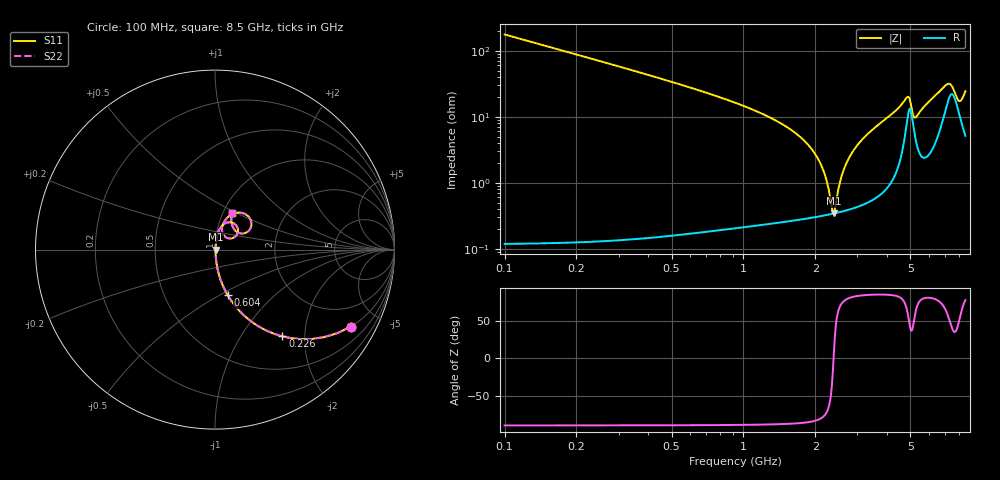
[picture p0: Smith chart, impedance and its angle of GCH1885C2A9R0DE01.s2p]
!Murata Part Number: GCH1885C2A9R0DE01
!These Parameters are Measured in Series Mode Connection
!Data Generated on Mar 13, 2026
!  o--ll--o
!Port1  Port2
!  o------o
!Operation Temp=25[degC], DC Bias Voltage=0[V]
!Freq. Start=100[MHz] Stop=9[GHz] 401[Steps]
# Hz S RI R 50
!Freq.(Hz) S11(Real) S11(Imag) S21(Real) S21(Imag) S12(Real) S12(Imag) S22(Real) S22(Imag)
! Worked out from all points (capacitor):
!   401 points, 100 MHz to 8.5 GHz, reference 50 ohm
!   read as one part in series: C = 9 pF near 142 MHz
!   lowest |Z| = 343 mohm at 2.389 GHz (marker M1)
!   series resonance near 2.385 GHz, so ESL is about 490 pH
!   S11 on the Smith chart (normalised r, x): 100 MHz: 1.00, -3.53; 226 MHz: 1.00, -1.55; 604 MHz: 1.00, -0.55; 8.5 GHz: 1.10, +0.48
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1e8  0.7569 -0.4286  0.2431 0.4286  0.2431 0.4286  0.7569 -0.4286
2.26e8  0.3757 -0.4835  0.6243 0.4835  0.6243 0.4835  0.3757 -0.4835
3.73e8  0.177 -0.3801  0.823 0.3801  0.823 0.3801  0.177 -0.3801
6.04e8  0.0713 -0.2542  0.9287 0.2542  0.9287 0.2542  0.0713 -0.2542
1.507e9  0.00758 -0.0706  0.9924 0.0706  0.9924 0.0706  0.00758 -0.0706
1.843e9  0.0044 -0.0391  0.9956 0.0391  0.9956 0.0391  0.0044 -0.0391
2.074e9  0.00353 -0.0212  0.9965 0.0212  0.9965 0.0212  0.00353 -0.0212
2.2e9  0.00336 -0.0123  0.9966 0.0123  0.9966 0.0123  0.00336 -0.0123
2.347e9  0.00337 -0.00244  0.9966 0.00244  0.9966 0.00244  0.00337 -0.00244
2.389e9  0.00341 0.00027  0.9966 -0.00027  0.9966 -0.00027  0.00341 0.00027
2.62e9  0.00391 0.0146  0.9961 -0.0146  0.9961 -0.0146  0.00391 0.0146
2.914e9  0.00514 0.0317  0.9949 -0.0317  0.9949 -0.0317  0.00514 0.0317
3.418e9  0.00887 0.0597  0.9911 -0.0597  0.9911 -0.0597  0.00887 0.0597
4.3e9  0.0261 0.1148  0.9739 -0.1148  0.9739 -0.1148  0.0261 0.1148
4.846e9  0.1044 0.1463  0.8956 -0.1463  0.8956 -0.1463  0.1044 0.1463
4.951e9  0.1283 0.1078  0.8717 -0.1078  0.8717 -0.1078  0.1283 0.1078
5.203e9  0.0587 0.0702  0.9413 -0.0702  0.9413 -0.0702  0.0587 0.0702
5.707e9  0.0414 0.1315  0.9586 -0.1315  0.9586 -0.1315  0.0414 0.1315
7.114e9  0.1771 0.1925  0.8229 -0.1925  0.8229 -0.1925  0.1771 0.1925
7.408e9  0.2026 0.137  0.7974 -0.137  0.7974 -0.137  0.2026 0.137
7.975e9  0.1161 0.1033  0.8839 -0.1033  0.8839 -0.1033  0.1161 0.1033
8.5e9  0.0954 0.2052  0.9046 -0.2052  0.9046 -0.2052  0.0954 0.2052
